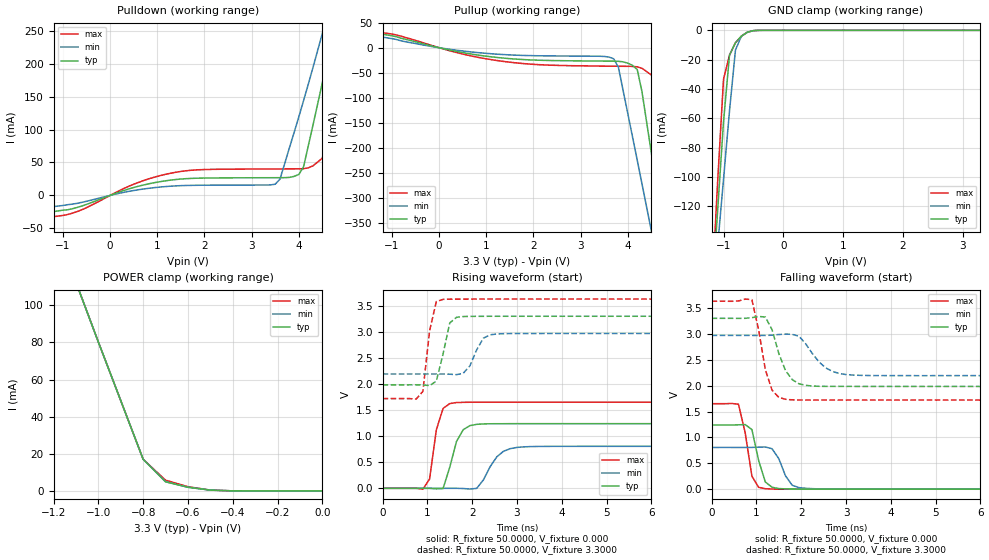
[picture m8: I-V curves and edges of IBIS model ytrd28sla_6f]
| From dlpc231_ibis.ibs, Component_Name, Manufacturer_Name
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| Model ytrd28sla_6f
[Model]   ytrd28sla_6f
Model_type   3-state
Polarity   Non-Inverting
Enable   Active-High
Vmeas = 1.5000V
Cref =50.0000pF
Rref = 0.5000k
Vref =  0.000V
C_comp   0.7000pF   0.7000pF   0.7000pF
[Temperature Range]   25.0000   0.1240k   -40.0000
[Voltage Range]   3.3000V   2.9700V   3.6300V
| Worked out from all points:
|   slope of the pulldown table from 0 to 0.495 V, typ, clamps not added: 41.7 ohm
|   slope of the pullup table from 0 to 0.495 V, typ, clamps not added: 51.3 ohm
|   GND clamp passes 1 mA (typ) near -0.57 V on its own axis
|   POWER clamp passes 1 mA (typ) near -0.54 V on its own axis
|   rising waveform, R_fixture 50.0000, V_fixture 0.000: 20-80 % time 270ps typ, 356ps min, 199ps max; typ from 0 V to 1.24 V
|   rising waveform, R_fixture 50.0000, V_fixture 3.3000: 20-80 % time 211ps typ, 257ps min, 179ps max; typ from 1.98 V to 3.3 V
|   falling waveform, R_fixture 50.0000, V_fixture 0.000: 20-80 % time 220ps typ, 272ps min, 199ps max; typ from 1.24 V to 0 V
|   falling waveform, R_fixture 50.0000, V_fixture 3.3000: 20-80 % time 323ps typ, 448ps min, 271ps max; typ from 3.3 V to 1.98 V
[Pulldown]
-3.3V     -36mA      -28mA      -45mA
-900mV    -21.82mA   -14.1mA    -29.04mA
1.4V      24.15mA    14.48mA    35.22mA
3.5V      26.85mA    17.01mA    40.14mA
3.6V      26.87mA    24.58mA    40.16mA
4V        31.8mA     119.2mA    40.29mA
4.1V      43.21mA    143.7mA    40.49mA
4.5V      171.5mA    246.1mA    56.57mA
4.7V      238.8mA    300.6mA    133.1mA
4.9V      308.6mA    358mA      217.1mA
5.1V      381.2mA    419.1mA    303.9mA
6.6V      1.058A     972.6mA    1.069A
[Pullup]
-3.3V     22mA       27.8mA     15mA
-1.5V     31.6mA     25.8mA     34mA
1.2V      -19.14mA   -12.66mA   -25.2mA
3.7V      -26.85mA   -22.07mA   -36.91mA
3.8V      -27.1mA    -38.84mA   -36.99mA
4.2V      -43.6mA    -224.9mA   -38.13mA
4.3V      -87.85mA   -271.8mA   -41.15mA
4.5V      -211mA     -366.2mA   -54.38mA
4.7V      -335.3mA   -461.2mA   -115.9mA
4.9V      -460.4mA   -556.8mA   -271.9mA
5.1V      -586.2mA   -652.9mA   -429mA
6.6V      -1.541A    -1.384A    -1.619A
[GND_clamp]
-3.3V     -1.515A    -1.204A    -1.847A
-1.2V     -185.5mA   -194.5mA   -182.5mA
-1.1V     -123.8mA   -147.9mA   -104.5mA
-1V       -62.37mA   -101.6mA   -33.38mA
-900mV    -16.91mA   -55.06mA   -16.91mA
-800mV    -8.434mA   -13.38mA   -8.434mA
-700mV    -3.946mA   -3.946mA   -3.946mA
-600mV    -1.264mA   -1.264mA   -1.264mA
-500mV    -213uA     -246.3uA   -196.1uA
-400mV    -14.84uA   -26.5uA    -10.46uA
3.3V      3.366nA    3.366nA    16.84nA
[POWER_clamp]
-3.3V     1.025A     838.2mA    1.218A
-1.1V     112.5mA    112.5mA    112.5mA
-1V       80.27mA    80.27mA    80.27mA
-800mV    17.07mA    17.07mA    17.07mA
-700mV    4.946mA    4.946mA    5.793mA
-600mV    1.98mA     1.98mA     2.27mA
-500mV    443.7uA    443.7uA    443.7uA
-400mV    34.77uA    34.77uA    34.77uA
0V        3.366nA    3.366nA    56.62nA
[Ramp]
dV/dt_r   0.7440/0.2366n   0.4834/0.3488n   0.9906/0.1802n
dV/dt_f   0.7896/0.3159n   0.4662/0.4456n   1.1454/0.2403n
R_load = 50.0000
[Rising Waveform]
R_fixture = 50.0000
V_fixture = 0.000
V_fixture_min = 0.000
V_fixture_max = 0.000
0s        0V         0V         0V
900ps     236.1uV    -2.06uV    -16.3mV
1.05ns    284.8uV    -4.441uV   179.6mV
1.2ns     -9.9mV     -2.908uV   1.12V
1.35ns    -4.975mV   76.88uV    1.532V
1.65ns    898.1mV    238.2uV    1.645V
2.1ns     1.227V     -1.393mV   1.651V
2.55ns    1.239V     604.1mV    1.651V
3.15ns    1.24V      795.2mV    1.651V
14.85ns   1.24V      805.7mV    1.651V
[Rising Waveform]
R_fixture = 50.0000
V_fixture = 3.3000
V_fixture_min = 2.9700
V_fixture_max = 3.6300
0s        1.984V     2.193V     1.721V
900ps     1.983V     2.193V     1.859V
1.05ns    1.97V      2.193V     3.021V
1.2ns     2.056V     2.193V     3.583V
1.35ns    2.575V     2.192V     3.624V
1.5ns     3.173V     2.189V     3.629V
1.65ns    3.28V      2.18V      3.629V
2.25ns    3.299V     2.88V      3.63V
2.55ns    3.3V       2.96V      3.63V
14.85ns   3.3V       2.97V      3.63V
[Falling Waveform]
R_fixture = 50.0000
V_fixture = 0.000
V_fixture_min = 0.000
V_fixture_max = 0.000
0s        1.24V      805.7mV    1.651V
600ps     1.243V     805.6mV    1.641V
750ps     1.248V     805.5mV    1.09V
900ps     1.151V     806.9mV    252.5mV
1.05ns    554.4mV    811.2mV    35.25mV
1.2ns     138mV      814.8mV    8.615mV
1.35ns    37.06mV    781.3mV    2.98mV
1.8ns     2.282mV    75.44mV    85.8uV
2.1ns     360uV      16.73mV    7.264uV
14.85ns   0V         0V         0V
[Falling Waveform]
R_fixture = 50.0000
V_fixture = 3.3000
V_fixture_min = 2.9700
V_fixture_max = 3.6300
0s        3.3V       2.97V      3.63V
900ps     3.313V     2.969V     3.661V
1.05ns    3.336V     2.969V     3.078V
1.2ns     3.326V     2.97V      2.306V
1.35ns    3.08V      2.974V     1.912V
1.65ns    2.291V     2.996V     1.736V
1.95ns    2.036V     2.955V     1.722V
2.55ns    1.986V     2.342V     1.721V
3.15ns    1.985V     2.204V     1.721V
14.85ns   1.984V     2.193V     1.721V
